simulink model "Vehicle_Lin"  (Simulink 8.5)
settings: Solver=ode3  StartTime=0.0  StopTime=1000  FixedStep=Ts  RelTol=1e-3
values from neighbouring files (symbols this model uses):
  ini = [wbo; atto; Hco]    [start.m]    (also in start1.m; start2.m; start3.m)
  wo = 0.0011    [start.m]    (also in start1.m; start2.m; start3.m)
undefined symbols (not defined in the file or in its folder): Linear2_LVLH

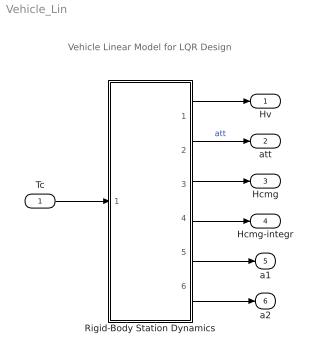
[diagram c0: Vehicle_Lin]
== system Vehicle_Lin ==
  note: Vehicle Linear Model for LQR Design
  Tc : Inport  PortDimensions=3
  Rigid-Body Station Dynamics : Subsystem
  Hv : Outport
  att : Outport  Port=2
  Hcmg : Outport  Port=3
  Hcmg-integr : Outport  Port=4
  a1 : Outport  Port=5
  a2 : Outport  Port=6
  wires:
  Rigid-Body Station Dynamics/3(Hcmg) -> Hcmg/1
  Rigid-Body Station Dynamics/4(Hintegr) -> Hcmg-integr/1
  Rigid-Body Station Dynamics/1(W-lv) -> Hv/1
  Rigid-Body Station Dynamics/2(atti-lv) -> att/1  "att"
  Tc/1 -> Rigid-Body Station Dynamics/1(Tcmg)
  Rigid-Body Station Dynamics/5(a1) -> a1/1
  Rigid-Body Station Dynamics/6(a2) -> a2/1

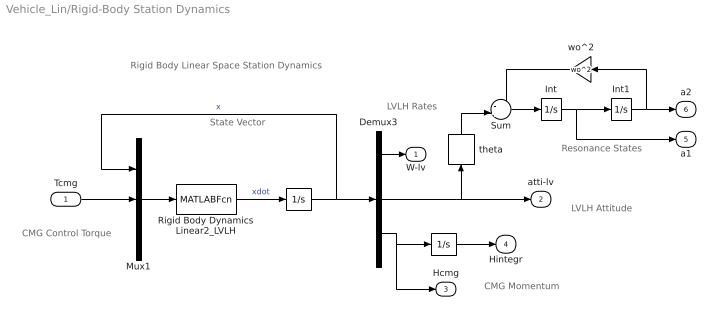
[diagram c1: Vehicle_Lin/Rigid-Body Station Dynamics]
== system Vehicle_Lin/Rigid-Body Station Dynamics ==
  note: Rigid Body Linear Space Station Dynamics
  note: State Vector
  note: CMG Momentum
  note: LVLH Attitude
  note: LVLH Rates
  note: Resonance States
  note: CMG Control Torque
  Tcmg : Inport  PortDimensions=3
  " " : Integrator
  "  " : Integrator  InitialCondition=ini
  Demux3 : Demux  Outputs=[3,3,3]
  Int : Integrator
  Int1 : Integrator
  Mux1 : Mux  Inputs=[9, 3, 3]
  Rigid Body Dynamics Linear2_LVLH : MATLABFcn  MATLABFcn=Linear2_LVLH( u(1:9), u(10:12), u(13:15) )  OutputDimensions=9
  Sum : Sum  Inputs=-+|
  theta : Selector  InputPortWidth=3  Indices=[2]
  wo^2 : Gain  Gain=wo^2
  W-lv : Outport
  atti-lv : Outport  Port=2
  Hcmg : Outport  Port=3
  Hintegr : Outport  Port=4
  a1 : Outport  Port=5
  a2 : Outport  Port=6
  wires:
  Rigid Body Dynamics Linear2_LVLH/1 -> "  "/1  "xdot"
  "  "/1 -> Demux3/1, Mux1/1  "x"
  Tcmg/1 -> Mux1/2
  Demux3/1 -> W-lv/1
  Demux3/2 -> atti-lv/1, theta/1
  Demux3/3 -> " "/1, Hcmg/1
  " "/1 -> Hintegr/1
  Mux1/1 -> Rigid Body Dynamics Linear2_LVLH/1
  Int/1 -> Int1/1, a1/1
  Sum/1 -> Int/1
  Int1/1 -> a2/1, wo^2/1
  wo^2/1 -> Sum/1
  theta/1 -> Sum/2
